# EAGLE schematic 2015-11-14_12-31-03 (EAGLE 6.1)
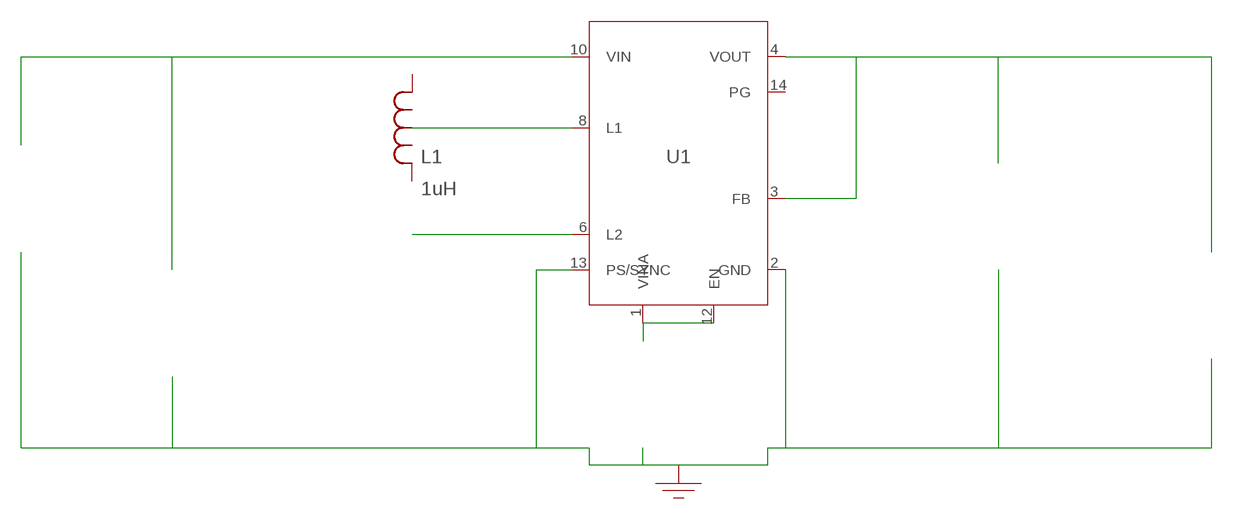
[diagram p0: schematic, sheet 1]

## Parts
CIN  22uF  GRM31CR61A226KE19LGRM31CR61A226KE19L  [1206_190]  (not placed on a sheet)
COUT  47uF  GRM31CR60J476ME19LGRM31CR60J476ME19L  [1206_190]  (not placed on a sheet)
CVINA  100nF  08053C104KAT2A08053C104KAT2A  [0805]  (not placed on a sheet)
GND  WB_GND  WB_GNDWB_GND  [WB_GND]
IOUT  WB_CURRENT_LOAD  WB_CURRENT_LOADWB_CURRENT_LOAD  [WB_CURRENT_LOAD]  (not placed on a sheet)
L1  1uH  MLP2520K1R0STMLP2520K1R0ST  [MLP2520K-S]
U1  TPS63021DSJR  TPS63021DSJRTPS63021DSJR  [R-PVSON-N14]
VIN  WB_BATTERY  WB_BATTERYWB_BATTERY  [WB_BATTERY]  (not placed on a sheet)

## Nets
0: Cin.2@2 Cout.2@2 CvinA.2@2 GND.1 Iout.-@2 U1.2(GND) U1.13(PS/SYNC) U1.15(PowerPAD) Vin.-@2
1: Cout.1@1 Iout.+@1 U1.3(FB) U1.4(VOUT) U1.5(VOUT)
2: L1.2 U1.8(L1) U1.9(L1)
3: CvinA.1@1 U1.1(VINA) U1.12(EN)
4: Cin.1@1 U1.10(VIN) U1.11(VIN) Vin.+@1
5: L1.1 U1.6(L2) U1.7(L2)
Unconnected: CIN.1 CIN.2 COUT.1 COUT.2 CVINA.1 CVINA.2 IOUT.1(+) IOUT.2(-) U1.14(PG) VIN.1(+) VIN.2(-)

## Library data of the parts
CIN = AcceleratedDesigns_Lib:GRM31CR61A226KE19L; Cap: 2.2E-5; ESR: 0.0; IRMS: 0.0; Manufacturer_Name: MuRata; Manufacturer_Part_Number: GRM31CR61A226KE19L; VDC: 10.0; Vendor: MuRata
COUT = AcceleratedDesigns_Lib:GRM31CR60J476ME19L; Cap: 4.7E-5; ESR: 0.0030; IRMS: 0.0; Manufacturer_Name: MuRata; Manufacturer_Part_Number: GRM31CR60J476ME19L; VDC: 6.3; Vendor: MuRata
CVINA = AcceleratedDesigns_Lib:08053C104KAT2A; Cap: 1.0E-7; ESR: 0.28; IRMS: 0.0; Manufacturer_Name: AVX; Manufacturer_Part_Number: 08053C104KAT2A; VDC: 25.0; Vendor: AVX
GND = AcceleratedDesigns_Lib:WB_GND; Manufacturer_Name: WB_GND; Manufacturer_Part_Number: WB_GND; PowerPortType: POWER_GROUND; Value: Value
IOUT = AcceleratedDesigns_Lib:WB_CURRENT_LOAD; Manufacturer_Name: WB_CURRENT_LOAD; Manufacturer_Part_Number: WB_CURRENT_LOAD; PowerPortType: POWER_GROUND; Value: Value
L1 = AcceleratedDesigns_Lib:MLP2520K1R0ST; Manufacturer_Name: TDK; Manufacturer_Part_Number: 'MLP2520K1R0ST'; Vendor: Gimme a name
U1 = AcceleratedDesigns_Lib:TPS63021DSJR; Datasheet_URL: http://www.ti.com/lit/ds/symlink/tps63020.pdf; Frequency: 2400000.0; Imax: 3.0; Manufacturer_Name: Texas Instruments; Manufacturer_Part_Number: TPS63021DSJR; Mktg_Package: TPS63020; NSID: TPS63021DSJR; Package: TPS63020; Vendor: Texas Instruments
VIN = AcceleratedDesigns_Lib:WB_BATTERY; Manufacturer_Name: WB_BATTERY; Manufacturer_Part_Number: WB_BATTERY; PowerPortType: POWER_GROUND; Value: Value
